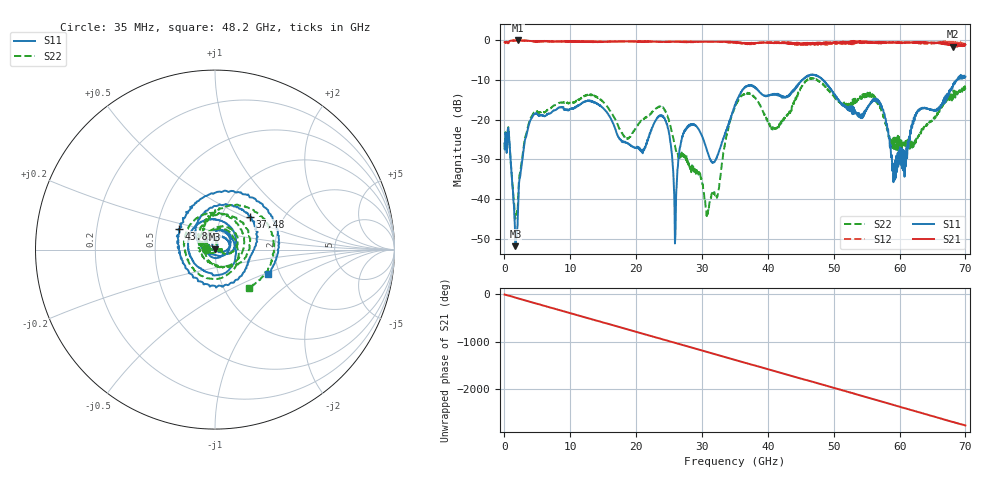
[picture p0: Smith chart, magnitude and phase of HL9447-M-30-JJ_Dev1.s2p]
! 8/12/2020 3:40:21 PM
! H:\PRODUCTION_DATA\TEMP_S2P.S2P
! CHANNEL.1
! TR.MEASUREMENT
! CORRECTED.DATA
# GHZ S RI R 50.0
! FREQ.GHZ  S11RE  S11IM  S21RE  S21IM  S12RE  S12IM  S22RE  S22IM
!; PortSelection: Port_12
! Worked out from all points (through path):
!   2000 points, 35 MHz to 70 GHz, reference 50 ohm
!   highest |S21| = -0.12 dB at 2.1 GHz (marker M1); lowest = -1.7 dB at 68.11 GHz (marker M2)
!   group delay of S21, straight-line fit = 110 ps
!   lowest |S11| = -51.8 dB at 1.68 GHz (marker M3), VSWR 1.01, Z = 50 + j0.255 ohm
!   |S11| at or under -10 dB: start of sweep to 45.27 GHz; 48.33 GHz to 68.75 GHz (20.42 GHz wide, 34.9 % of centre)
!   |S22| runs from -44.9 to -9.5 dB; largest |S21 - S12| = 0.14
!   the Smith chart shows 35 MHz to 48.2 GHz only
!   S11 on the Smith chart (normalised r, x): 35 MHz: 0.90, +0.01; 37.48 GHz: 1.36, +0.53; 43.85 GHz: 0.65, +0.16; 48.2 GHz: 1.73, -0.53
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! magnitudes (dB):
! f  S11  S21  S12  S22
! 35 MHz  -26.0  -0.5  -0.5  -25.8
! 805 MHz  -26.9  -0.3  -0.3  -26.8
! 1.68 GHz  -51.8  -0.1  -0.1  -44.9
! 2.1 GHz  -41.1  -0.1  -0.2  -39.7
! 4.235 GHz  -19.3  -0.3  -0.3  -18.9
! 11.72 GHz  -15.9  -0.4  -0.4  -14.5
! 20.89 GHz  -27.8  -0.4  -0.4  -20.1
! 23.38 GHz  -19.2  -0.5  -0.5  -16.9
! 24.89 GHz  -22.3  -0.4  -0.4  -19.7
! 25.93 GHz  -50.0  -0.4  -0.4  -26.8
! 27.65 GHz  -22.0  -0.5  -0.6  -28.9
! 30.84 GHz  -28.2  -0.4  -0.4  -43.7
! 35.03 GHz  -16.4  -0.6  -0.6  -16.6
! 37.48 GHz  -11.5  -0.9  -0.9  -13.8
! 40.84 GHz  -13.7  -0.8  -0.5  -22.2
! 43.85 GHz  -12.8  -0.9  -0.7  -15.8
! 46.69 GHz  -8.8  -1.0  -1.1  -9.6
! 48.2 GHz  -9.8  -0.8  -1.0  -10.9
! 58.34 GHz  -24.3  -0.6  -0.7  -24.3
! 59.29 GHz  -33.3  -0.6  -0.6  -27.3
! 68.11 GHz  -11.6  -1.7  -0.5  -14.9
! 70 GHz  -9.2  -1.2  -1.2  -12.7
